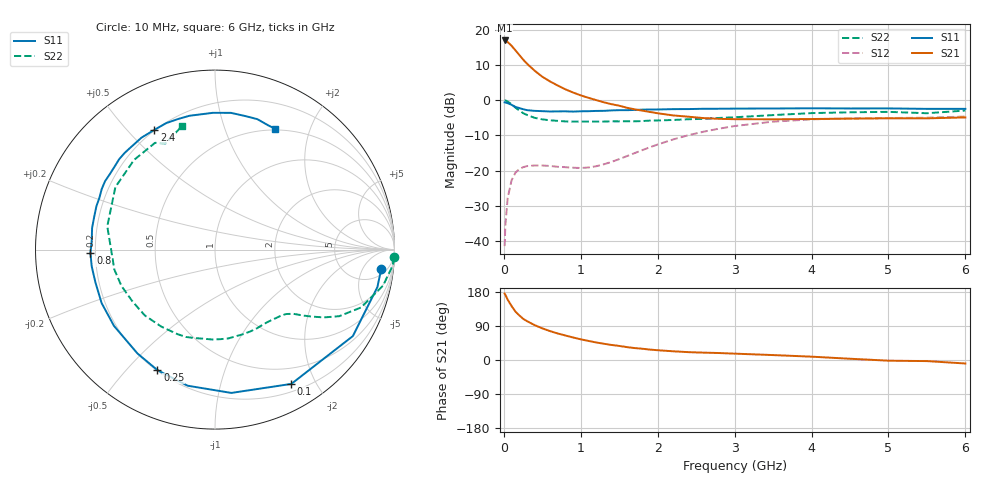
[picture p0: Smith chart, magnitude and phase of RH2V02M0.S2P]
! SIEMENS Small Signal Semiconductors
! BFR106
! Si NPN RF Bipolar Junction Transistor in SOT23
! VCE = 2 V  IC = 2 mA
! Common Emitter S-Parameters:  August  1996
# GHz  S  MA  R  50
!  f  S11  S21  S12  S22
! GHz  MAG  ANG  MAG  ANG  MAG  ANG  MAG  ANG
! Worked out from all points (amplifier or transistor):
!   36 points, 10 MHz to 6 GHz, reference 50 ohm
!   highest |S21| = 17.0 dB at 10 MHz (marker M1)
!   |S21| within 3 dB of that: start of sweep to 157.9 MHz
!   unconditionally stable (mu >= 1): 779.8 MHz to 2.234 GHz; 2.764 GHz to end of sweep
!   at 250 MHz: K = 0.33, MSG = 15.3 dB, |S12| = -19.1 dB
!   at 1.4 GHz: K = 1.30, MAG = 4.9 dB, |S12| = -17.6 dB
!   at 6 GHz: K = 1.02, MAG = -1.0 dB, |S12| = -4.6 dB
!   S11 on the Smith chart (normalised r, x): 10 MHz: 8, -13; 100 MHz: 0.29, -1.68; 250 MHz: 0.20, -0.61; 800 MHz: 0.18, -0.01; 2.4 GHz: 0.20, +0.60; 6 GHz: 0.49, +1.51
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0.01  0.9325 -6.6  7.07 175.2  0.0084 86.9  0.9977 -2.5
0.02  0.9286 -13.0  7.065 171.9  0.0166 81.9  0.9941 -5.1
0.05  0.9067 -32.1  6.706 159.2  0.0408 72.7  0.9575 -12.1
0.1  0.8607 -60.4  5.956 142.6  0.0722 58.2  0.8754 -21.6
0.15  0.8037 -83.5  5.125 127.9  0.0929 46.5  0.7852 -28.2
0.2  0.7735 -101.4  4.411 117.9  0.1047 38.9  0.7149 -31.9
0.25  0.7443 -115.5  3.791 108.9  0.1115 33.2  0.6558 -34.7
0.3  0.7222 -126.7  3.312 102.6  0.1155 29.5  0.6169 -36.6
0.4  0.7054 -142.9  2.63 92.1  0.118 24.7  0.5617 -39.5
0.5  0.6984 -154.8  2.156 83.5  0.1179 22.4  0.5337 -42.3
0.6  0.6908 -164.6  1.849 76.3  0.1161 22.0  0.5182 -45.7
0.8  0.6944 -178.4  1.428 64.7  0.1114 25.4  0.4994 -53.4
1.1  0.6973 164.9  1.081 50.3  0.1105 38.5  0.4966 -66.8
1.6  0.7214 144.2  0.78 34.0  0.1603 59.3  0.501 -92.0
2.2  0.7462 123.3  0.608 23.0  0.2764 59.6  0.5231 -124.9
2.4  0.7477 116.9  0.582 20.7  0.3183 56.5  0.5361 -136.8
3  0.7591 100.8  0.537 16.8  0.4291 43.5  0.5717 -168.8
3.5  0.7621 90.9  0.535 13.0  0.4955 32.0  0.614 167.8
4.5  0.7629 77.1  0.547 3.3  0.55 12.0  0.673 132.1
5  0.7641 72.0  0.553 -1.8  0.5577 4.5  0.6823 119.3
5.5  0.7529 66.7  0.552 -2.9  0.564 1.1  0.6525 115.0
6  0.7525 63.4  0.569 -9.2  0.5856 -6.4  0.7127 104.9
